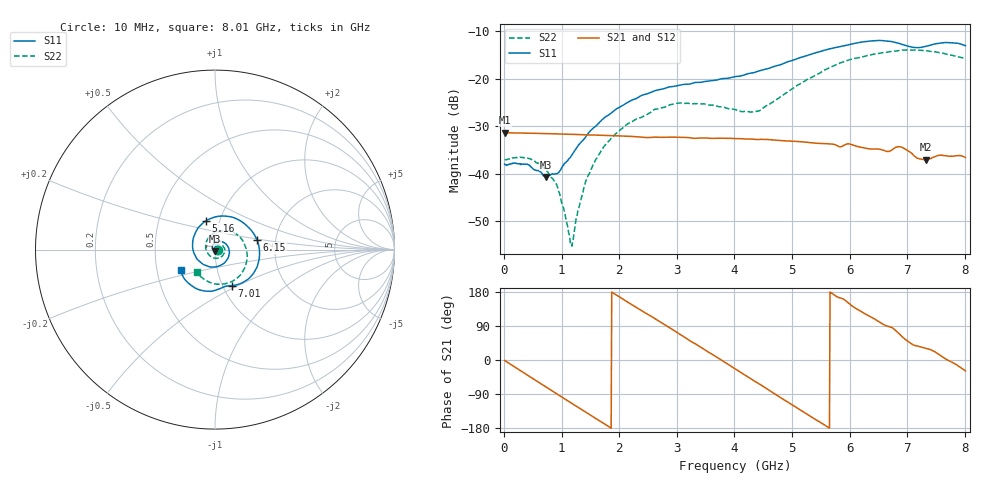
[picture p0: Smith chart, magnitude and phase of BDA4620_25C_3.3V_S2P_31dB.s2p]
!Agilent Technologies,E5071B,MY42404982,A.09.10
!Date: Wed May 06 08:55:37 2026
!Data & Calibration Information:
!Freq	S11:SOLT2(ON)	S21:SOLT2(ON)	S12:SOLT2(ON)	S22:SOLT2(ON)
# Hz S RI R 50
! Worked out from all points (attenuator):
!   801 points, 10 MHz to 8.01 GHz, reference 50 ohm
!   highest |S21| = -31.36 dB at 20 MHz (marker M1); lowest = -37.1 dB at 7.33 GHz (marker M2)
!   lowest |S11| = -40.7 dB at 720 MHz (marker M3), VSWR 1.02, Z = 49.9 - j0.918 ohm
!   |S11| at or under -10 dB: start of sweep to end of sweep
!   |S22| runs from -55.3 to -13.9 dB; largest |S21 - S12| = 0.00018
!   S11 on the Smith chart (normalised r, x): 10 MHz: 1.03, -0.00; 5.16 GHz: 0.86, +0.29; 6.15 GHz: 1.60, +0.19; 7.01 GHz: 1.10, -0.46; 8.01 GHz: 0.66, -0.16
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1e7  0.0126 -0.000746  0.027 -0.000548  0.0271 -0.000545  0.014 -0.000497
2e7  0.0124 -0.000779  0.027 -0.000985  0.027 -0.00108  0.014 -0.000326
4.4e8  0.00867 -0.00864  0.0194 -0.0182  0.0194 -0.0182  0.0134 -0.00507
7.2e8  -0.000716 -0.00919  0.0089 -0.0249  0.00888 -0.0249  0.0085 -0.00721
9.3e8  -0.00851 -0.00529  -0.000298 -0.0263  -0.000302 -0.0263  0.00361 -0.00618
1.16e9  -0.0144 0.00467  -0.0101 -0.0239  -0.0101 -0.0239  -0.00139 -0.00116
1.2e9  -0.015 0.00683  -0.0116 -0.0231  -0.0117 -0.0232  -0.00201 -1.33e-06
1.35e9  -0.0154 0.0155  -0.0169 -0.0194  -0.0169 -0.0194  -0.00346 0.00453
1.53e9  -0.0118 0.0269  -0.0217 -0.0134  -0.0218 -0.0134  -0.00332 0.0112
1.77e9  0.000705 0.0398  -0.0249 -0.00388  -0.025 -0.00384  0.000753 0.0204
2.14e9  0.0328 0.0455  -0.0222 0.0111  -0.0222 0.0111  0.0164 0.0288
2.68e9  0.076 0.00858  -0.00556 0.0235  -0.00558 0.0235  0.0441 0.0196
3.08e9  0.0739 -0.0449  0.01 0.0219  0.0101 0.0219  0.055 -0.00706
4.01e9  -0.0645 -0.0828  0.0215 -0.00917  0.0216 -0.0092  -0.0101 -0.0463
4.43e9  -0.1207 -0.00903  0.0104 -0.0203  0.0104 -0.0204  -0.0444 -0.0116
5.16e9  -0.0499 0.1611  -0.0149 -0.0156  -0.0149 -0.0157  -0.0096 0.0889
5.35e9  0.00581 0.1832  -0.0186 -0.01  -0.0186 -0.0101  0.0229 0.1016
6.15e9  0.2336 0.0549  -0.0129 0.0142  -0.0129 0.0143  0.1635 0.0319
6.68e9  0.1958 -0.1544  0.000522 0.0171  0.000614 0.0171  0.1702 -0.0898
7.01e9  0.0925 -0.2005  0.0113 0.0132  0.0113 0.0133  0.1219 -0.1599
7.33e9  0.0247 -0.2185  0.0121 0.00712  0.0121 0.00715  0.0453 -0.1923
8.01e9  -0.1908 -0.1162  0.013 -0.00707  0.013 -0.00708  -0.1012 -0.1273
